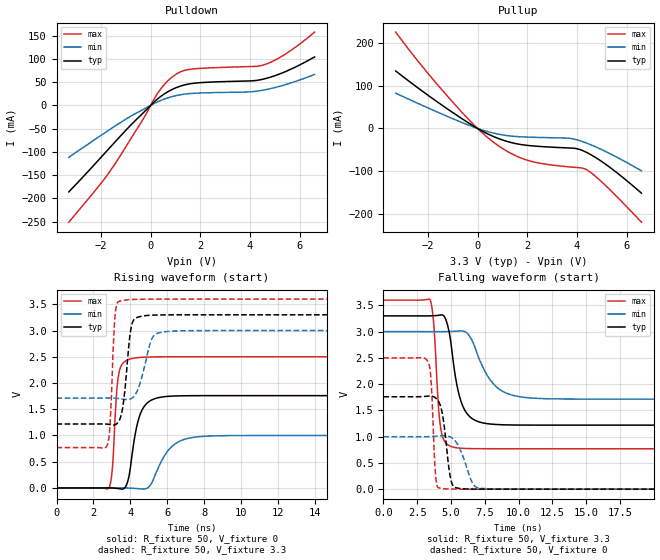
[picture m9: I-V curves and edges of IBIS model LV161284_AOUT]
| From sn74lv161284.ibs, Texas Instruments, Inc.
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[Model]   LV161284_AOUT
Model_type  Output
Vref =   0
Rref =   500
Cref =   50p
Vmeas =   1.4
| variable   typ   min   max
C_comp   4.18pF   2.71pF   5.56pF
| C_pullup   4.22pF   2.71pF   5.35pF
| C_pulldown   4.14pF   3.01pF   5.56pF
[Temperature Range]   40   100   -40
| Ambient temperature   25   85   -40
[Voltage range]   3.3   3   3.6
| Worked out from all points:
|   slope of the pulldown table from 0 to 0.495 V, typ, clamps not added: 21.9 ohm
|   slope of the pullup table from 0 to 0.495 V, typ, clamps not added: 32.9 ohm
|   rising waveform, R_fixture 50, V_fixture 0: 20-80 % time 550ps typ, 992ps min, 250ps max; typ from 0 V to 1.76 V
|   falling waveform, R_fixture 50, V_fixture 3.3: 20-80 % time 855ps typ, 1.56ns min, 396ps max; typ from 3.3 V to 1.22 V
|   rising waveform, R_fixture 50, V_fixture 3.3: 20-80 % time 338ps typ, 559ps min, 204ps max; typ from 1.22 V to 3.3 V
|   falling waveform, R_fixture 50, V_fixture 0: 20-80 % time 490ps typ, 844ps min, 256ps max; typ from 1.76 V to 0 V
[Pulldown]
| LV161284_AOUT
|   Voltage   I(typ)   I(min)   I(max)
-3.3V     -186.1mA   -111.8mA   -251.2mA
-1.685V   -93.22mA   -53.35mA   -145mA
-375mV    -20.06mA   -11mA      -35.79mA
275mV     13.64mA    7.441mA    25.46mA
565mV     25.07mA    13.75mA    45.69mA
880mV     34.49mA    18.95mA    61.51mA
1.23V     41.8mA     22.92mA    72.59mA
1.62V     46.54mA    25.38mA    77.55mA
3.95V     52.36mA    28.8mA     83.24mA
4.555V    56.56mA    32.9mA     86.99mA
5.45V     72.99mA    44.81mA    111mA
6.6V      104mA      66.36mA    157.4mA
[Pullup]
| LV161284_AOUT
|   Voltage   I(typ)   I(min)   I(max)
-3.3V     133.9mA    82.14mA    224.4mA
-2.27V    88.81mA    54.94mA    147.4mA
-1.18V    44.1mA     27.2mA     73mA
-170mV    5.902mA    3.555mA    9.673mA
595mV     -17.64mA   -10.14mA   -29.89mA
1.31V     -32.09mA   -17.38mA   -56.97mA
2.02V     -39.45mA   -20.04mA   -74.15mA
3.695V    -45.44mA   -22.81mA   -89.41mA
4.035V    -47.63mA   -26.96mA   -91.04mA
4.385V    -55.61mA   -33.93mA   -95.92mA
5.135V    -82.36mA   -53mA      -131.7mA
6.6V      -150.6mA   -98.47mA   -218.2mA
[Ramp]
| LV161284_AOUT
| variable   typ   min   max
dV/dt_r   1.07/5.59E-10   0.61/9.95E-10   1.51/2.62E-10
dV/dt_f   1.26/8.62E-10   0.78/1.56E-09   1.71/4.00E-10
R_load = 50
[Rising Waveform]
| LV161284_AOUT
R_fixture =   50
C_fixture =   0
L_fixture =   0
V_fixture =   0
V_fixture_min = 0
V_fixture_max = 0
|   Time   V(typ)   V(min)   V(max)
0s        104.2pV    215.6pV    40.77pV
2.845ns   1.154mV    13.28uV    5.576mV
3.025ns   10.39uV    195.2uV    380.5mV
3.25ns    -7.45mV    538.7uV    1.8V
3.4ns     -14.09mV   720uV      2.223V
3.86ns    131.1mV    -1.219mV   2.442V
4.41ns    1.268V     -13.53mV   2.485V
6.38ns    1.752V     829.8mV    2.5V
8.22ns    1.76V      989.4mV    2.501V
70ns      1.76V      999.8mV    2.501V
[Falling Waveform]
| LV161284_AOUT
R_fixture =   50
C_fixture =   0
L_fixture =   0
V_fixture =   3.3
V_fixture_min = 3
V_fixture_max = 3.6
|   Time   V(typ)   V(min)   V(max)
0s        3.3V       3V         3.6V
3.45ns    3.3V       3V         3.61V
3.735ns   3.304V     3V         3.106V
4.265ns   3.319V     3V         1.122V
4.805ns   3.06V      3.002V     839.1mV
5.37ns    2.073V     3.008V     790mV
6.66ns    1.328V     2.775V     771.6mV
8.29ns    1.233V     1.964V     769.6mV
10.88ns   1.22V      1.736V     769.5mV
70ns      1.219V     1.714V     769.4mV
[Rising Waveform]
| LV161284_AOUT
R_fixture =   50
C_fixture =   0
L_fixture =   0
V_fixture =   3.3
V_fixture_min = 3
V_fixture_max = 3.6
|   Time   V(typ)   V(min)   V(max)
0s        1.219V     1.714V     769.4mV
2.745ns   1.216V     1.715V     812.5mV
2.9ns     1.208V     1.715V     1.23V
3.2ns     1.209V     1.711V     3.386V
3.55ns    1.46V      1.695V     3.57V
3.8ns     2.246V     1.685V     3.585V
4.205ns   3.214V     1.752V     3.594V
5.2ns     3.294V     2.869V     3.599V
6.265ns   3.299V     2.99V      3.6V
70ns      3.3V       3V         3.6V
[Falling Waveform]
| LV161284_AOUT
R_fixture =   50
C_fixture =   0
L_fixture =   0
V_fixture =   0
V_fixture_min = 0
V_fixture_max = 0
|   Time   V(typ)   V(min)   V(max)
0s        1.76V      999.8mV    2.501V
3.345ns   1.773V     1.001V     2.405V
3.545ns   1.772V     1.003V     1.985V
3.855ns   1.739V     1.01V      275.4mV
4.11ns    1.655V     1.015V     21.33mV
5.01ns    158.8mV    984.8mV    2.253mV
5.77ns    9.911mV    699.5mV    383.2uV
6.68ns    1.435mV    82mV       56.24uV
7.77ns    244.7uV    6.417mV    7.265uV
70ns      104pV      215.5pV    40.74pV
